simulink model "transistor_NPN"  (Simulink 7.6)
settings: Solver=ode15s  StartTime=0.0  StopTime=0.04  RelTol=1e-3
InitFcn:
  | Rc=100e3;
  | Re=10e3;
  | Rb=22e3;
StopFcn:
  | delete *.mat
libraries: fl_lib x10, nesl_utility x3, elec_lib x1, AppliElectrical_lib x1

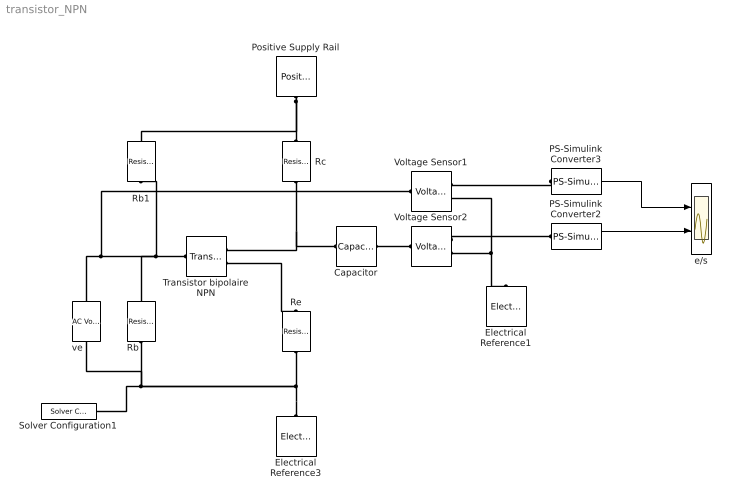
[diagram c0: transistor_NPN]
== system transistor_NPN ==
  Capacitor : fl_lib/Electrical/Electrical Elements/Capacitor  DialogController=NetworkEngine.DynNeDlgSource  SystemSampleTime=-1  c=47e-3 F  v0=0 V  r=1e-6 Ohm  g=0 1/Ohm  i_Log=off  v_Log=off  vc_Log=off  LocalVarNames=|i|v|vc  LocalVarDescs=|i|v|Internal variable for voltage across capacitor term  LocalVarLogging=[0 0 0]
  Electrical Reference1 : fl_lib/Electrical/Electrical Elements/Electrical Reference  DialogController=NetworkEngine.DynNeDlgSource  SystemSampleTime=-1  i_Log=off  LocalVarNames=|i  LocalVarDescs=|i  LocalVarLogging=0
  Electrical Reference3 : fl_lib/Electrical/Electrical Elements/Electrical Reference  DialogController=NetworkEngine.DynNeDlgSource  SystemSampleTime=-1  i_Log=off  LocalVarNames=|i  LocalVarDescs=|i  LocalVarLogging=0
  PS-Simulink Converter2 : nesl_utility/PS-Simulink Converter  DialogController=NetworkEngine.DynNeUtilDlgSource  SystemSampleTime=-1  PhysicalDomain=network_engine_domain  LeftPortType=input  RightPortType=output  SubClassName=ps_output  Unit=1  AffineConversion=off
  PS-Simulink Converter3 : nesl_utility/PS-Simulink Converter  DialogController=NetworkEngine.DynNeUtilDlgSource  SystemSampleTime=-1  PhysicalDomain=network_engine_domain  LeftPortType=input  RightPortType=output  SubClassName=ps_output  Unit=1  AffineConversion=off
  Positive Supply Rail : elec_lib/Sources/Positive Supply Rail  DialogController=NetworkEngine.DynNeDlgSource  SystemSampleTime=-1  v0=15 V  current_Log=off  voltage_Log=off  power_Log=off  LocalVarNames=|current|voltage|power  LocalVarDescs=|Current (A)|Voltage (V)|Power (W)  LocalVarLogging=[0 0 0]
  Rb : fl_lib/Electrical/Electrical Elements/Resistor  DialogController=NetworkEngine.DynNeDlgSource  SystemSampleTime=-1  R=22 kOhm  i_Log=off  v_Log=off  LocalVarNames=|i|v  LocalVarDescs=|i|v  LocalVarLogging=[0 0]
  Rb1 : fl_lib/Electrical/Electrical Elements/Resistor  DialogController=NetworkEngine.DynNeDlgSource  SystemSampleTime=-1  R=100 kOhm  i_Log=off  v_Log=off  LocalVarNames=|i|v  LocalVarDescs=|i|v  LocalVarLogging=[0 0]
  Rc : fl_lib/Electrical/Electrical Elements/Resistor  DialogController=NetworkEngine.DynNeDlgSource  SystemSampleTime=-1  R=Rc kOhm  i_Log=off  v_Log=off  LocalVarNames=|i|v  LocalVarDescs=|i|v  LocalVarLogging=[0 0]
  Re : fl_lib/Electrical/Electrical Elements/Resistor  DialogController=NetworkEngine.DynNeDlgSource  SystemSampleTime=-1  R=Re kOhm  i_Log=off  v_Log=off  LocalVarNames=|i|v  LocalVarDescs=|i|v  LocalVarLogging=[0 0]
  Solver Configuration1 : nesl_utility/Solver Configuration  DialogController=NetworkEngine.DynNeUtilDlgSource  SystemSampleTime=-1  PhysicalDomain=network_engine_domain  LeftPortType=input  RightPortType=generic  SubClassName=solver  Accelerate=off  Profile=off  ResidualTolerance=1e-9  MaxNonlinIter=3  MaxModeIter=2  DoFixedCost=off  UseLocalSampling=off  DoDC=off  LinearAlgebra=Sparse  LocalSolverSampleTime=.001  LocalSolverChoice=NE_BACKWARD_EULER_ADVANCER  UseLocalSolver=off
  Transistor bipolaire NPN : AppliElectrical_lib/Transistor bipolaire NPN  DialogController=NetworkEngine.DynNeDlgSource  SystemSampleTime=-1  s=1e-6 1/Ohm  h21=200  h12=1e-4  h11=1000 Ohm  Ib_Log=off  Vbe_Log=off  Ic_Log=off  Vce_Log=off  LocalVarNames=|Ib|Vbe|Ic|Vce  LocalVarDescs=|courant d'entrée du transistor|tension, Base-Emetteur|courant Collecteur-Emetteur|tension Collecteur-Emetteur  LocalVarLogging=[0 0 0 0]
  Voltage Sensor1 : fl_lib/Electrical/Electrical Sensors/Voltage Sensor  DialogController=NetworkEngine.DynNeDlgSource  SystemSampleTime=-1  i1_Log=off  v1_Log=off  LocalVarNames=|i1|v1  LocalVarDescs=|i1|v1  LocalVarLogging=[0 0]
  Voltage Sensor2 : fl_lib/Electrical/Electrical Sensors/Voltage Sensor  DialogController=NetworkEngine.DynNeDlgSource  SystemSampleTime=-1  i1_Log=off  v1_Log=off  LocalVarNames=|i1|v1  LocalVarDescs=|i1|v1  LocalVarLogging=[0 0]
  e/s : Scope  NumInputPorts=2
  ve : fl_lib/Electrical/Electrical Sources/AC Voltage Source  DialogController=NetworkEngine.DynNeDlgSource  SystemSampleTime=-1  amp=10 mV  shift=0 rad  omega=60 Hz  i_Log=off  v_Log=off  LocalVarNames=|i|v  LocalVarDescs=|i|v  LocalVarLogging=[0 0]
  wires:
  PS-Simulink Converter2/1 -> e/s/2
  PS-Simulink Converter3/1 -> e/s/1
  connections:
  Electrical Reference3/LConn1 -- Solver Configuration1/RConn1 -- ve/RConn1 -- Rb/LConn1 -- Re/LConn1
  Transistor bipolaire NPN/LConn1 -- ve/LConn1 -- Voltage Sensor1/LConn1 -- Rb/RConn1 -- Rb1/LConn1
  Voltage Sensor2/RConn2 -- Electrical Reference1/LConn1 -- Voltage Sensor1/RConn2
  Voltage Sensor2/RConn1 -- PS-Simulink Converter2/LConn1
  PS-Simulink Converter3/LConn1 -- Voltage Sensor1/RConn1
  Rc/LConn1 -- Transistor bipolaire NPN/RConn1 -- Capacitor/LConn1
  Transistor bipolaire NPN/RConn2 -- Re/RConn1
  Capacitor/RConn1 -- Voltage Sensor2/LConn1
  Positive Supply Rail/RConn1 -- Rc/RConn1 -- Rb1/RConn1
